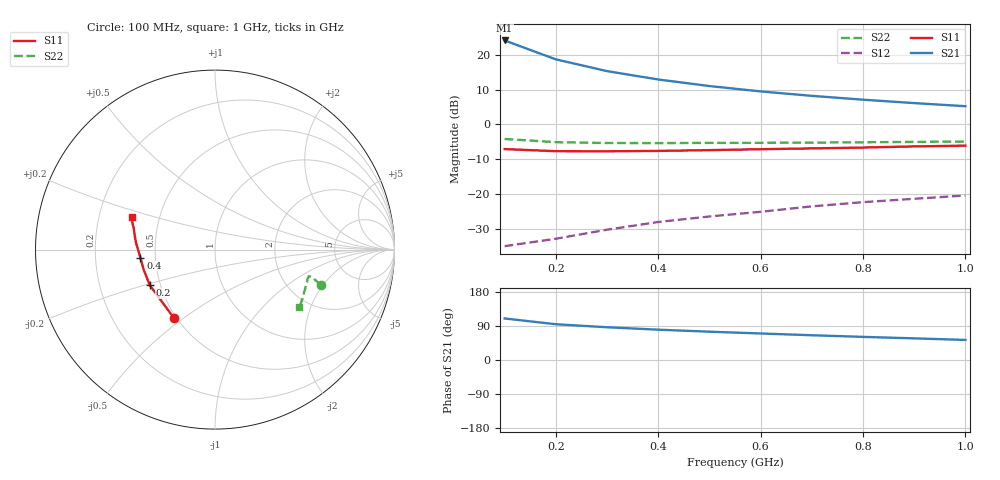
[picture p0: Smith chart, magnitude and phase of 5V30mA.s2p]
#  HZ  S  MA  R  50.0000
! Device:15GN03CA
! "! Bias:VCE=5V, IC=30mA  "
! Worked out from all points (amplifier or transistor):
!   10 points, 100 MHz to 1 GHz, reference 50 ohm
!   highest |S21| = 24.1 dB at 100 MHz (marker M1)
!   |S21| within 3 dB of that: start of sweep to 155.4 MHz
!   unconditionally stable (mu >= 1): 135.2 MHz to end of sweep
!   at 200 MHz: K = 1.37, MAG = 22.1 dB, |S12| = -32.8 dB
!   at 600 MHz: K = 1.53, MAG = 12.9 dB, |S12| = -25.0 dB
!   at 1 GHz: K = 1.26, MAG = 9.7 dB, |S12| = -20.4 dB
!   S11 on the Smith chart (normalised r, x): 100 MHz: 0.48, -0.46; 200 MHz: 0.44, -0.21; 400 MHz: 0.41, -0.05; 1 GHz: 0.35, +0.17
1e8  0.444 -121.2  16.03 109.6  0.018 56.5  0.62 -18.3
2e8  0.414 -151.5  8.59 94.4  0.023 58.5  0.558 -15.7
3e8  0.413 -164.9  5.826 86.4  0.031 69.3  0.543 -15.9
4e8  0.418 -173.8  4.42 80.0  0.04 71.4  0.541 -17.6
5e8  0.429 179.9  3.56 74.7  0.048 75.9  0.545 -20.0
6e8  0.442 175.0  2.98 70.0  0.056 78.1  0.546 -22.4
7e8  0.454 170.1  2.575 65.3  0.067 79.8  0.55 -25.1
8e8  0.467 165.6  2.268 61.0  0.077 82.0  0.556 -27.9
9e8  0.485 161.8  2.027 57.1  0.086 84.0  0.563 -31.5
1e9  0.497 158.3  1.829 53.0  0.096 85.0  0.57 -34.4
